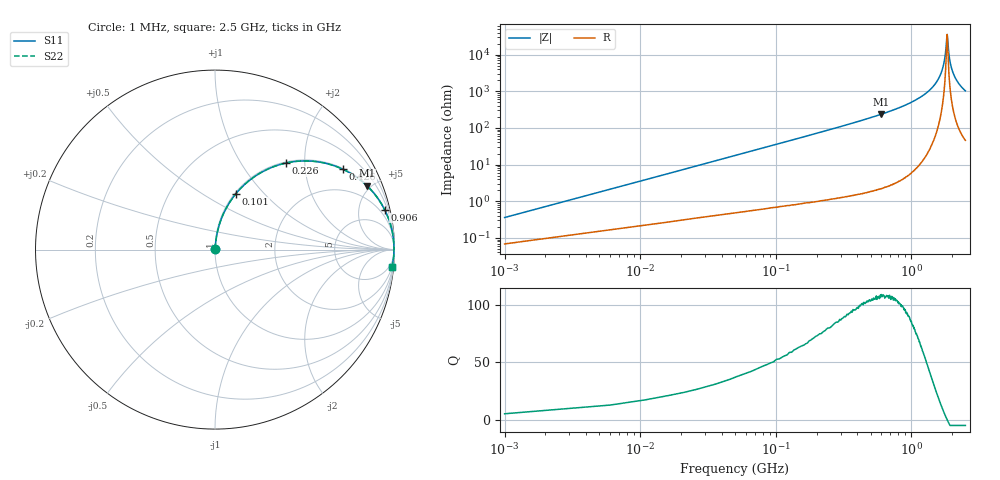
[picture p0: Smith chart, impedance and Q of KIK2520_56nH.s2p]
!version-2
!date-01.2022
!Series
# MHz S RI R 50
!Freq ReS11 ImS11 ReS21 ImS21 ReS12 ImS12 ReS22 ImS22
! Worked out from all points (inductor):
!   501 points, 1 MHz to 2.5 GHz, reference 50 ohm
!   read as one part in series: L = 56 nH near 11 MHz
!   highest Q = 108 at 601 MHz (marker M1), where L = 62.7 nH
!   self-resonance near 1.83 GHz
!   S11 on the Smith chart (normalised r, x): 1 MHz: 1.00, +0.01; 101 MHz: 1.01, +0.71; 226 MHz: 1.02, +1.61; 426 MHz: 1.03, +3.17; 906 MHz: 1.09, +8.43; 2.5 GHz: 2, -20
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1  0.00069 0.00351  0.9993 -0.00351  0.9993 -0.00351  0.00069 0.00351
16  0.00584 0.0558  0.9942 -0.0558  0.9942 -0.0558  0.00584 0.0558
31  0.0154 0.107  0.9846 -0.107  0.9846 -0.107  0.0154 0.107
61  0.0487 0.2033  0.9513 -0.2033  0.9513 -0.2033  0.0487 0.2033
101  0.1174 0.3125  0.8826 -0.3125  0.8826 -0.3125  0.1174 0.3125
226  0.396 0.4826  0.604 -0.4826  0.604 -0.4826  0.396 0.4826
421  0.7079 0.4497  0.2921 -0.4497  0.2921 -0.4497  0.7079 0.4497
426  0.7132 0.4473  0.2868 -0.4473  0.2868 -0.4473  0.7132 0.4473
601  0.8465 0.3559  0.1535 -0.3559  0.1535 -0.3559  0.8465 0.3559
836  0.9302 0.2498  0.0698 -0.2498  0.0698 -0.2498  0.9302 0.2498
906  0.9446 0.2234  0.0554 -0.2234  0.0554 -0.2234  0.9446 0.2234
1255  0.9836 0.1179  0.0163 -0.1179  0.0163 -0.1179  0.9836 0.1179
1505  0.9939 0.061  0.00609 -0.061  0.00609 -0.061  0.9939 0.061
1670  0.9966 0.0287  0.00337 -0.0287  0.00337 -0.0287  0.9966 0.0287
1760  0.9972 0.0126  0.00284 -0.0126  0.00284 -0.0126  0.9972 0.0126
1790  0.9972 0.00734  0.00278 -0.00734  0.00278 -0.00734  0.9972 0.00734
1825  0.9972 0.00138  0.00279 -0.00138  0.00279 -0.00138  0.9972 0.00138
1835  0.9972 -0.000306  0.0028 0.000306  0.0028 0.000306  0.9972 -0.000306
1885  0.997 -0.00858  0.00296 0.00858  0.00296 0.00858  0.997 -0.00858
1925  0.9968 -0.015  0.00319 0.015  0.00319 0.015  0.9968 -0.015
2085  0.9951 -0.0396  0.00487 0.0396  0.00487 0.0396  0.9951 -0.0396
2500  0.9864 -0.0957  0.0136 0.0957  0.0136 0.0957  0.9864 -0.0957
